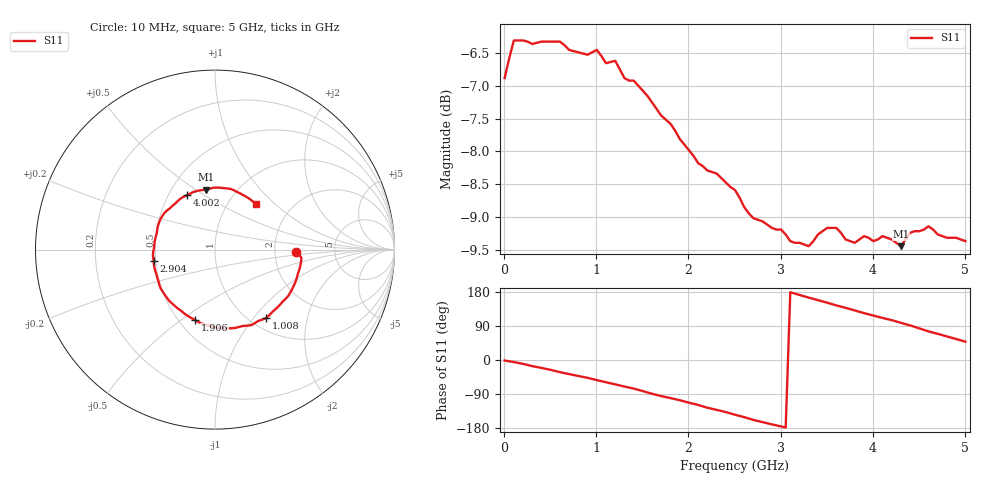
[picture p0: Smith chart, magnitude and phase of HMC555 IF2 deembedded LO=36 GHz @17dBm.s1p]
!Hittite Microwave Corporation
!20 Alpha Road
!Chelmsford, MA 01824
!Tel: 978-250-3343
!Fax: 978-250-3373
!Device: HMC555, 32-38GHz, I/Q Mixer
!Misc: IF2 Return Loss with LO = 36 GHz @ 17 dBm, Data includes one K connector, Room
# MHZ S MA R 50
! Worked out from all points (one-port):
!   101 points, 10 MHz to 5 GHz, reference 50 ohm
!   lowest |S11| = -9.4 dB at 4.301 GHz (marker M1), VSWR 2.02, Z = 36.7 + j27.6 ohm
!   |S11| at or under -10 dB: nowhere
!   S11 on the Smith chart (normalised r, x): 10 MHz: 2.65, -0.07; 1.008 GHz: 1.18, -1.16; 1.906 GHz: 0.60, -0.56; 2.904 GHz: 0.49, -0.07; 4.002 GHz: 0.62, +0.42; 5 GHz: 1.33, +0.77
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10  0.453 -1.4
109.8  0.484 -5.5
209.6  0.484 -10.2
459.1  0.483 -23.4
658.7  0.48 -34.6
1008  0.476 -52.9
1257.5  0.46 -67.2
1407.2  0.451 -75.3
1556.9  0.439 -85.6
1706.6  0.424 -95.2
1906.2  0.407 -106.1
2205.6  0.385 -126.0
2355.3  0.38 -134.5
2505  0.372 -144.5
2704.6  0.354 -158.1
2904.2  0.348 -169.9
3153.7  0.339 175.2
3303.4  0.337 164.6
3503  0.348 151.2
3602.8  0.348 144.0
3752.5  0.34 134.2
3902.2  0.343 123.8
4002  0.34 117.3
4101.8  0.343 111.0
4301.4  0.337 98.1
4401.2  0.345 91.3
4650.7  0.347 72.2
5000  0.34 48.3
